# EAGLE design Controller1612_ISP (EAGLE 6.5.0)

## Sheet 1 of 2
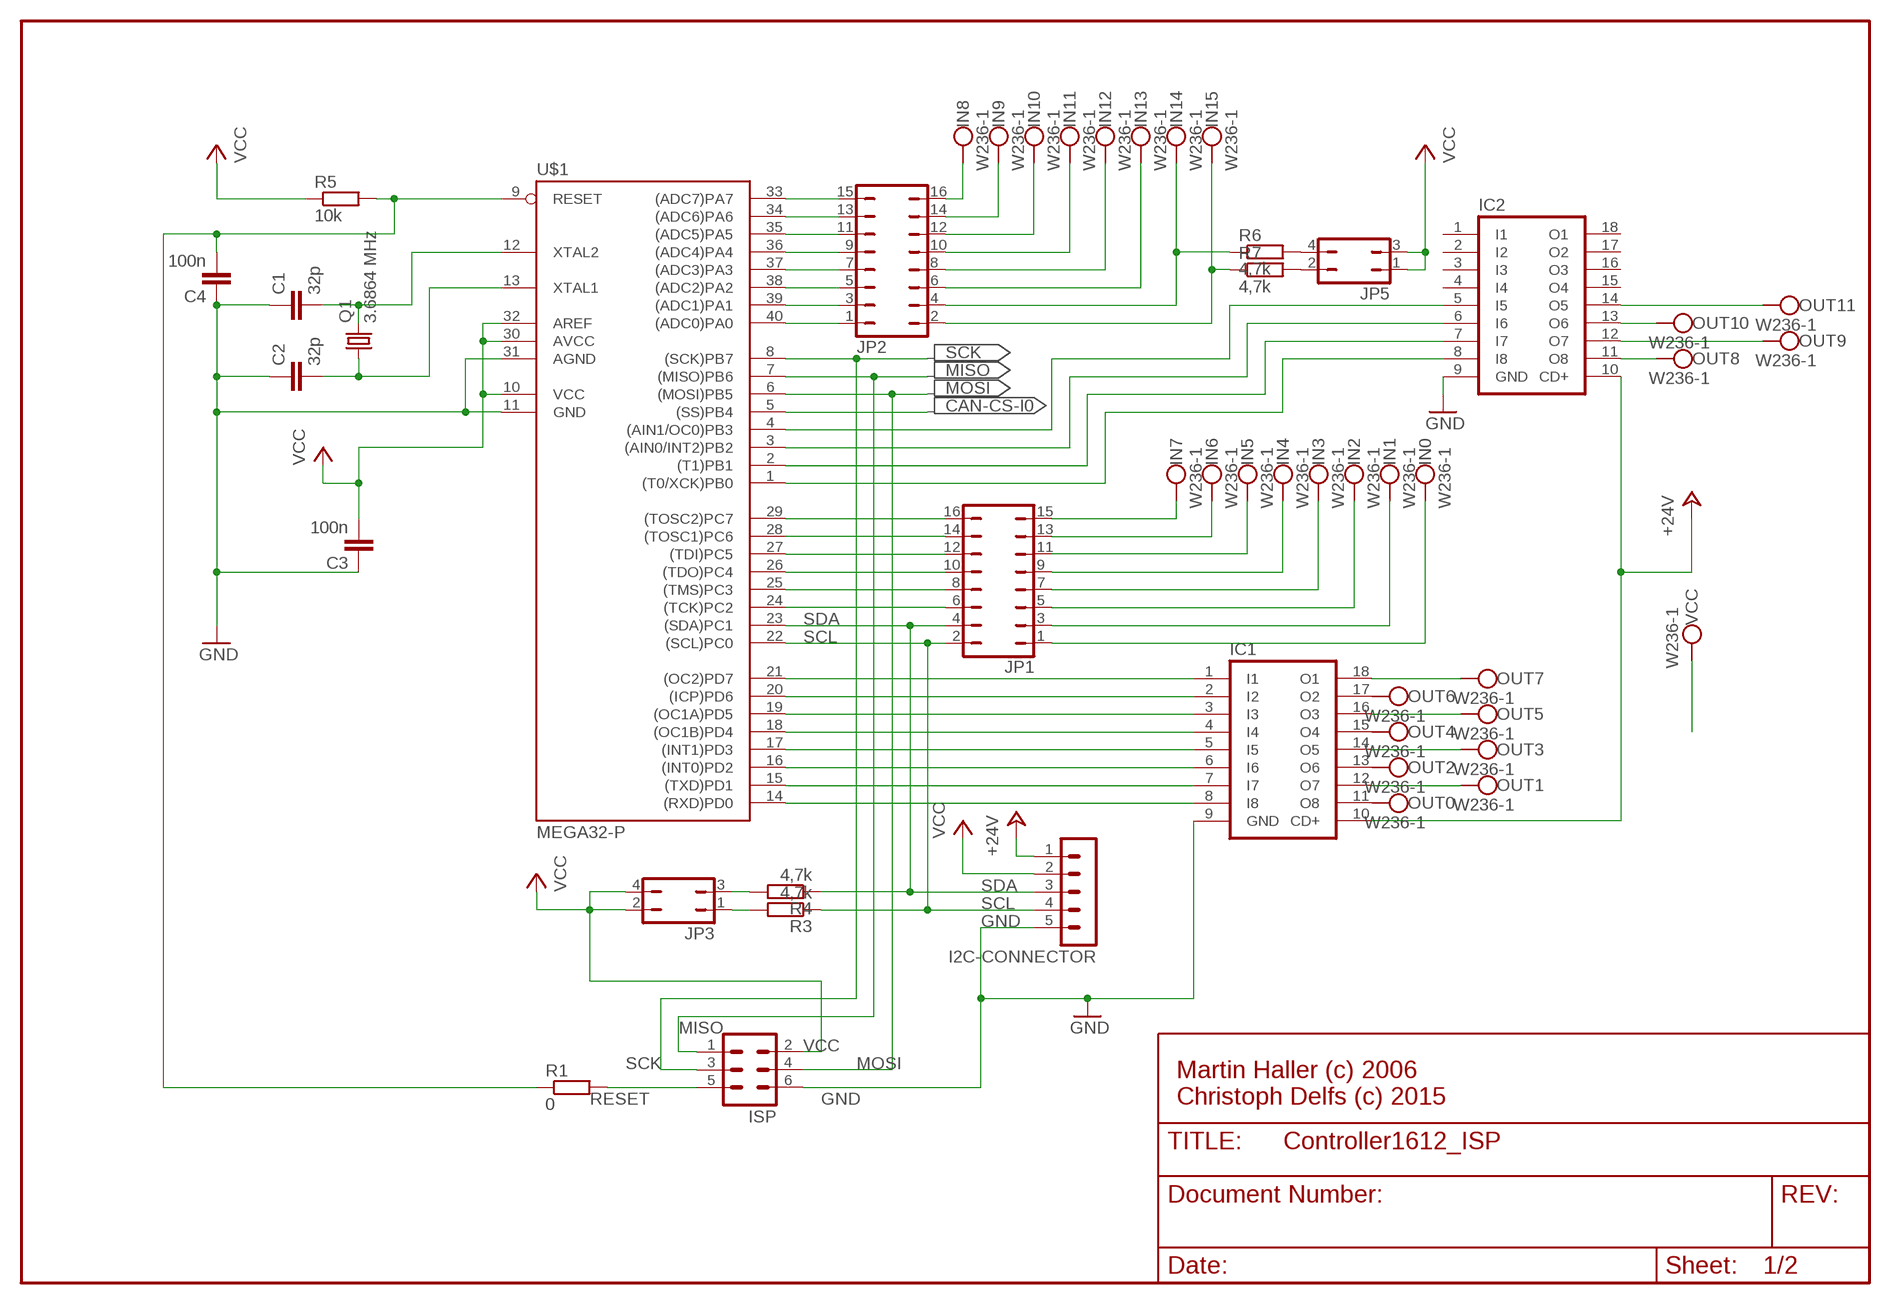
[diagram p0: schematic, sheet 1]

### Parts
C1  32p  C-EU025-024X044  [C025-024X044]
C2  32p  C-EU025-024X044  [C025-024X044]
C3  100n  C-EU050-025X075  [C050-025X075]
C4  100n  C-EU050-025X075  [C050-025X075]
I2C-CONNECTOR  MA05-1  [MA05-1]
IC1  ULN2803A  [DIL18]
IC2  ULN2803A  [DIL18]
IN0  W236-1  [W236-1]
IN1  W236-1  [W236-1]
IN2  W236-1  [W236-1]
IN3  W236-1  [W236-1]
IN4  W236-1  [W236-1]
IN5  W236-1  [W236-1]
IN6  W236-1  [W236-1]
IN7  W236-1  [W236-1]
IN8  W236-1  [W236-1]
IN9  W236-1  [W236-1]
IN10  W236-1  [W236-1]
IN11  W236-1  [W236-1]
IN12  W236-1  [W236-1]
IN13  W236-1  [W236-1]
IN14  W236-1  [W236-1]
IN15  W236-1  [W236-1]
ISP  ML6  [ML6]
JP1  JP8Q  [JP8Q]
JP2  JP8Q  [JP8Q]
JP3  JP2Q  [JP2Q]
JP5  JP2Q  [JP2Q]
OUT0  W236-1  [W236-1]
OUT1  W236-1  [W236-1]
OUT2  W236-1  [W236-1]
OUT3  W236-1  [W236-1]
OUT4  W236-1  [W236-1]
OUT5  W236-1  [W236-1]
OUT6  W236-1  [W236-1]
OUT7  W236-1  [W236-1]
OUT8  W236-1  [W236-1]
OUT9  W236-1  [W236-1]
OUT10  W236-1  [W236-1]
OUT11  W236-1  [W236-1]
Q1  3.6864 MHz  CRYTALHC49U70  [HC49U70]
R1  0  R-EU_0204/2V  [0204V]
R3  4,7k  R-EU_0204/7  [0204/7]
R4  4,7k  R-EU_0204/7  [0204/7]
R5  10k  R-EU_0207/12  [0207/12]
R6  4,7k  R-EU_0207/2V  [0207/2V]
R7  4,7k  R-EU_0207/2V  [0207/2V]
U$1  MEGA32-P  [DIL40]
VCC  W236-1  [W236-1]

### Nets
+24V: I2C-CONNECTOR.1 IC1.10(CD+) IC2.10(CD+) ; also sheet 2
CAN-CS-I0: U$1.5((SS)PB4) ; also sheet 2
GND: C1.1 C2.1 C3.1 C4.1 I2C-CONNECTOR.5 IC1.9(GND) IC2.9(GND) ISP.6 U$1.11(GND) U$1.31(AGND) ; also sheet 2
INPUT2: IN3.1(KL1) JP1.7
MISO: ISP.1 U$1.7((MISO)PB6) ; also sheet 2
MOSI: ISP.4 U$1.6((MOSI)PB5) ; also sheet 2
N$1: C1.2 Q1.2 U$1.12(XTAL2)
N$2: C2.2 Q1.1 U$1.13(XTAL1)
N$3: IN0.1(KL1) JP1.1
N$4: IN1.1(KL1) JP1.3
N$5: IN2.1(KL1) JP1.5
N$6: JP2.1 U$1.40((ADC0)PA0)
N$7: IN4.1(KL1) JP1.9
N$8: IN5.1(KL1) JP1.11
N$9: IN6.1(KL1) JP1.13
N$10: IN7.1(KL1) JP1.15
N$11: JP2.3 U$1.39((ADC1)PA1)
N$12: JP2.5 U$1.38((ADC2)PA2)
N$13: JP3.1 R3.2
N$14: JP2.7 U$1.37((ADC3)PA3)
N$15: JP2.9 U$1.36((ADC4)PA4)
N$16: JP2.11 U$1.35((ADC5)PA5)
N$17: JP2.13 U$1.34((ADC6)PA6)
N$18: IC1.1(I1) U$1.21((OC2)PD7)
N$19: IC1.2(I2) U$1.20((ICP)PD6)
N$20: IC1.3(I3) U$1.19((OC1A)PD5)
N$21: IC1.4(I4) U$1.18((OC1B)PD4)
N$22: IC1.5(I5) U$1.17((INT1)PD3)
N$23: IC1.6(I6) U$1.16((INT0)PD2)
N$24: IC1.7(I7) U$1.15((TXD)PD1)
N$25: IC1.8(I8) U$1.14((RXD)PD0)
N$26: IC1.11(O8) OUT0.1(KL1)
N$27: IC1.12(O7) OUT1.1(KL1)
N$28: IC1.13(O6) OUT2.1(KL1)
N$29: IC1.14(O5) OUT3.1(KL1)
N$30: IC1.15(O4) OUT4.1(KL1)
N$31: IC1.16(O3) OUT5.1(KL1)
N$32: IC1.17(O2) OUT6.1(KL1)
N$33: IC1.18(O1) OUT7.1(KL1)
N$34: IC2.8(I8) U$1.1((T0/XCK)PB0)
N$35: IC2.7(I7) U$1.2((T1)PB1)
N$36: IC2.6(I6) U$1.3((AIN0/INT2)PB2)
N$37: IC2.5(I5) U$1.4((AIN1/OC0)PB3)
N$38: IC2.11(O8) OUT8.1(KL1)
N$39: IC2.12(O7) OUT9.1(KL1)
N$40: IC2.13(O6) OUT10.1(KL1)
N$41: IC2.14(O5) OUT11.1(KL1)
N$42: JP2.15 U$1.33((ADC7)PA7)
N$52: IN8.1(KL1) JP2.16
N$53: IN9.1(KL1) JP2.14
N$54: IN10.1(KL1) JP2.12
N$55: IN11.1(KL1) JP2.10
N$56: IN12.1(KL1) JP2.8
N$57: IN13.1(KL1) JP2.6
N$58: IN14.1(KL1) JP2.4 R6.1
N$59: IN15.1(KL1) JP2.2 R7.1
N$60: JP3.3 R4.2
N$61: ISP.5 R1.2
N$62: JP1.6 U$1.24((TCK)PC2)
N$63: JP1.8 U$1.25((TMS)PC3)
N$64: JP1.10 U$1.26((TDO)PC4)
N$65: JP1.12 U$1.27((TDI)PC5)
N$66: JP1.14 U$1.28((TOSC1)PC6)
N$67: JP1.16 U$1.29((TOSC2)PC7)
N$68: JP5.4 R6.2
N$70: JP5.2 R7.2
RESET: C4.2 R1.1 R5.2 U$1.9(RESET)
SCK: ISP.3 U$1.8((SCK)PB7) ; also sheet 2
SCL: I2C-CONNECTOR.4 JP1.2 R3.1 U$1.22((SCL)PC0)
SDA: I2C-CONNECTOR.3 JP1.4 R4.1 U$1.23((SDA)PC1)
VCC: C3.2 I2C-CONNECTOR.2 ISP.2 JP3.2 JP3.4 JP5.1 JP5.3 R5.1 U$1.10(VCC) U$1.30(AVCC) U$1.32(AREF) VCC.1(KL1) ; also sheet 2
Unconnected: IC2.1(I1) IC2.2(I2) IC2.3(I3) IC2.4(I4) IC2.15(O4) IC2.16(O3) IC2.17(O2) IC2.18(O1) IN0.2(KL2) IN1.2(KL2) IN2.2(KL2) IN3.2(KL2) IN4.2(KL2) IN5.2(KL2) IN6.2(KL2) IN7.2(KL2) IN8.2(KL2) IN9.2(KL2) IN10.2(KL2) IN11.2(KL2) IN12.2(KL2) IN13.2(KL2) IN14.2(KL2) IN15.2(KL2) OUT0.2(KL2) OUT1.2(KL2) OUT2.2(KL2) OUT3.2(KL2) OUT4.2(KL2) OUT5.2(KL2) OUT6.2(KL2) OUT7.2(KL2) OUT8.2(KL2) OUT9.2(KL2) OUT10.2(KL2) OUT11.2(KL2) VCC.2(KL2)

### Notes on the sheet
- Martin Haller (c) 2006
  Christoph Delfs (c) 2015

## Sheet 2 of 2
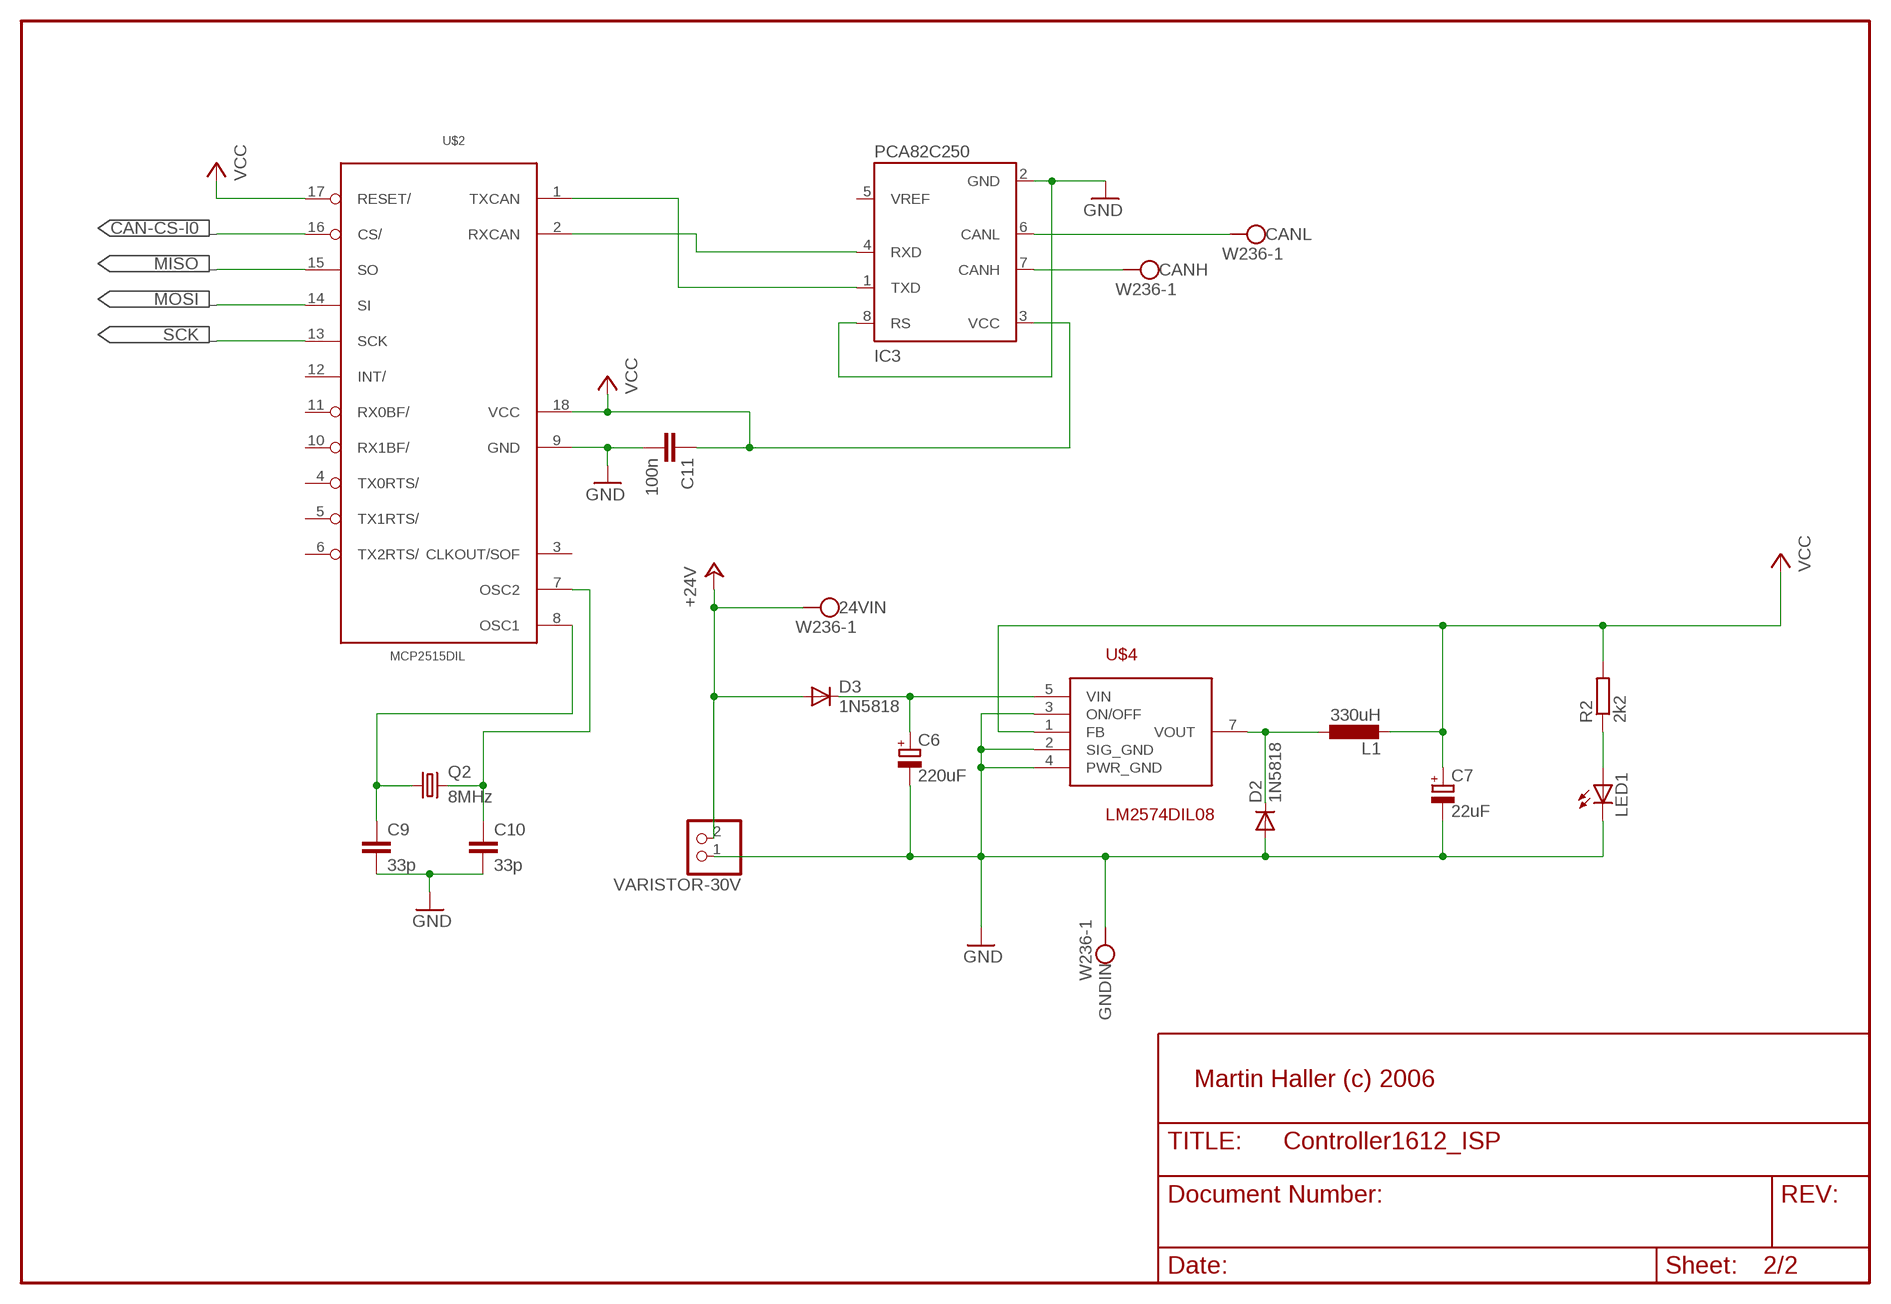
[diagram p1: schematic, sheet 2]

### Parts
24VIN  W236-1  [W236-1]
C6  220uF  CPOL-EUE22-10AXIAL  [E22-10]
C7  22uF  CPOL-EUE15-6AXIAL  [E15-6]
C9  33p  C-EU025-024X044  [C025-024X044]
C10  33p  C-EU025-024X044  [C025-024X044]
C11  100n  C-EU050-025X075  [C050-025X075]
CANH  W236-1  [W236-1]
CANL  W236-1  [W236-1]
D2  1N5818  1N4148  [DO35-10]
D3  1N5818  1N4148  [DO35-10]
GNDIN  W236-1  [W236-1]
IC3  PCA82C250  [DIL08]
L1  330uH  L-EU2200-12.7  [2200-12.7]
LED1  LED3MM  [LED3MM]
Q2  8MHz  CRYTALHC49U70  [HC49U70]
R2  2k2  R-EU_0207/2V  [0207/2V]
U$2  MCP2515DIL  [DIL18]
U$4  LM2574DIL08  [DIL08]
VARISTOR-30V  PINHD-1X2  [1X02]

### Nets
+24V: 24VIN.1(KL1) D3.A VARISTOR-30V.2 ; also sheet 1
CAN-CS-I0: U$2.16(CS/) ; also sheet 1
GND: C6.- C7.- C9.2 C10.2 C11.2 D2.A GNDIN.1(KL1) IC3.2(GND) IC3.8(RS) LED1.K(C) U$2.9(GND) U$4.2(SIG_GND) U$4.3(ON/OFF) U$4.4(PWR_GND) VARISTOR-30V.1 ; also sheet 1
MISO: U$2.15(SO) ; also sheet 1
MOSI: U$2.14(SI) ; also sheet 1
N$43: C6.+ D3.C U$4.5(VIN)
N$44: IC3.4(RXD) U$2.2(RXCAN)
N$45: IC3.1(TXD) U$2.1(TXCAN)
N$46: C9.1 Q2.1 U$2.8(OSC1)
N$47: C10.1 Q2.2 U$2.7(OSC2)
N$48: CANH.1(KL1) IC3.7(CANH)
N$49: CANL.1(KL1) IC3.6(CANL)
N$50: D2.C L1.1 U$4.7(VOUT)
N$51: LED1.A R2.1
SCK: U$2.13(SCK) ; also sheet 1
VCC: C7.+ C11.1 IC3.3(VCC) L1.2 R2.2 U$2.17(RESET/) U$2.18(VCC) U$4.1(FB) ; also sheet 1
Unconnected: 24VIN.2(KL2) CANH.2(KL2) CANL.2(KL2) GNDIN.2(KL2) IC3.5(VREF) U$2.3(CLKOUT/SOF) U$2.4(TX0RTS/) U$2.5(TX1RTS/) U$2.6(TX2RTS/) U$2.10(RX1BF/) U$2.11(RX0BF/) U$2.12(INT/)

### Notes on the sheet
- Martin Haller (c) 2006

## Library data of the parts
24VIN CANH CANL GNDIN IN0 IN1-IN15 OUT0 OUT1-OUT11 VCC = con-wago-508:W236-1: WAGO SREW CLAMP
C1-C4 C9-C11 = rcl:C-EU: CAPACITOR, European symbol
C6 C7 = rcl:CPOL-EU: POLARIZED CAPACITOR, European symbol
D2 D3 = diode:1N4148: DIODE
I2C-CONNECTOR = con-lstb:MA05-1: PIN HEADER
IC1 IC2 = uln-udn:ULN2803A: DRIVER ARRAY
IC3 = micro-philips:PCA82C250: CAN CONTROLLER INTERFACE
ISP = con-ml:ML6: HARTING; OC_FARNELL: unknown; OC_NEWARK: unknown
JP1 JP2 = jumper:JP8Q: JUMPER
JP3 JP5 = jumper:JP2Q: JUMPER
L1 = rcl:L-EU: INDUCTOR, European symbol
LED1 = led:LED: LED
Q1 Q2 = crystal:CRYTAL: CRYSTAL
R1 = resistor:R-EU_: RESISTOR, European symbol
R2-R7 = rcl:R-EU_: RESISTOR, European symbol
U$1 = avr:MEGA32-P: MICROCONTROLLER 32 Kbytes FLASH 2 Kbytes SRAM 1 Kbytes EEPROM USART 8-channel 10 bit ADC
U$2 = MCP2515_MT:MCP2515*: MCP2515 Standalone CAN-Controller by Microchip Eagle-Lib. by MartinThomas
U$4 = hausbus-bauteile:LM2574
VARISTOR-30V = pinhead:PINHD-1X2: PIN HEADER

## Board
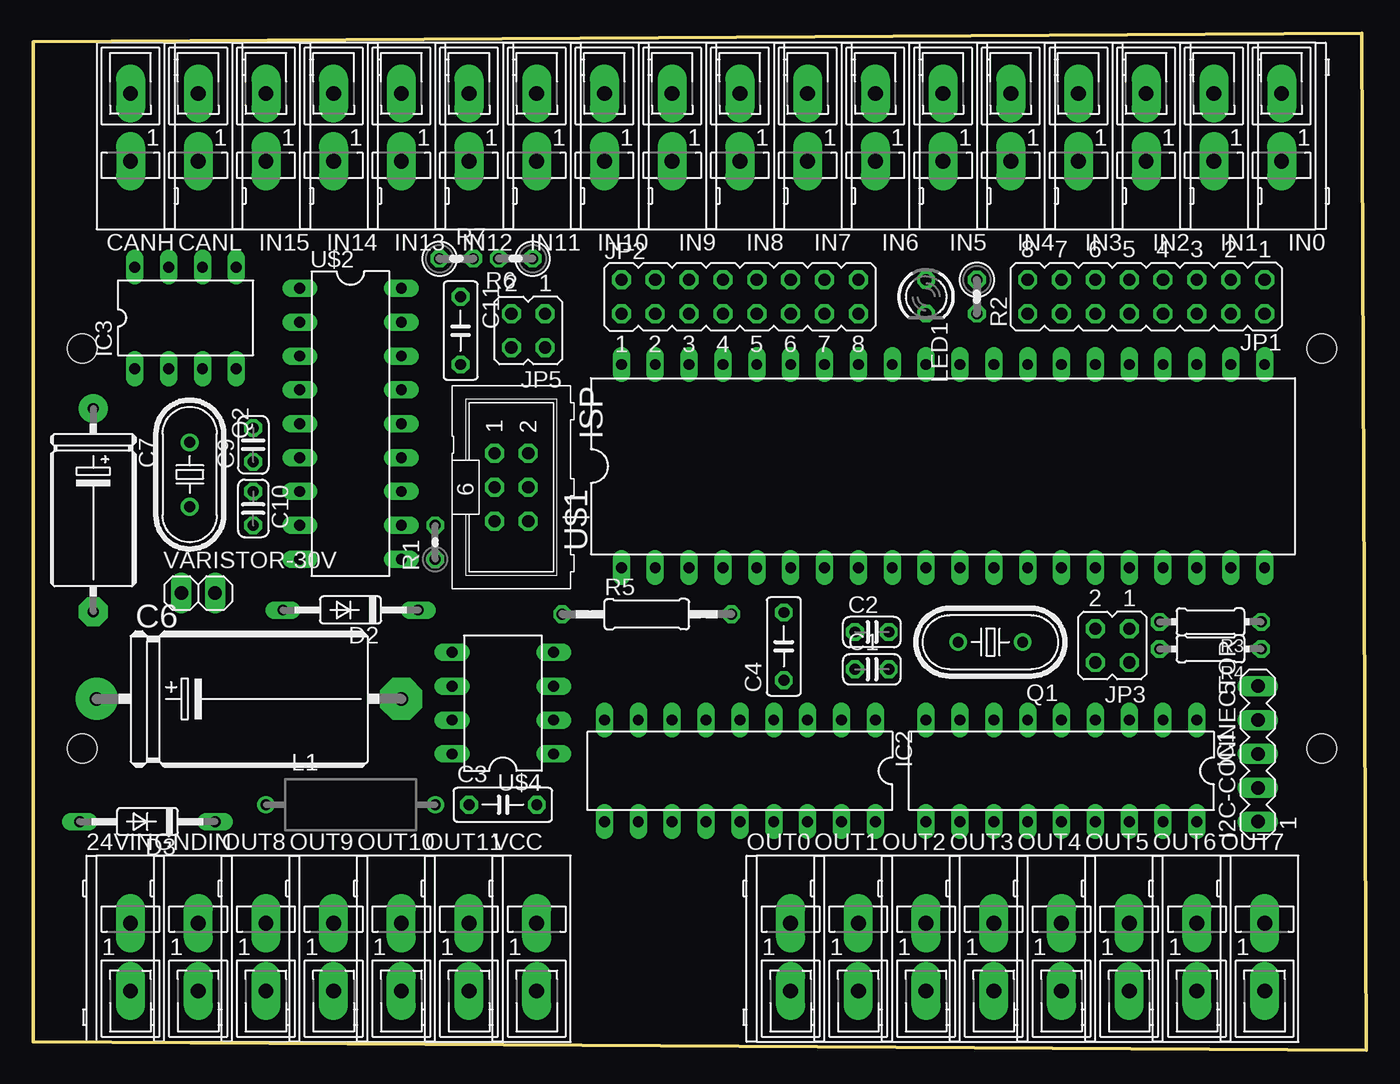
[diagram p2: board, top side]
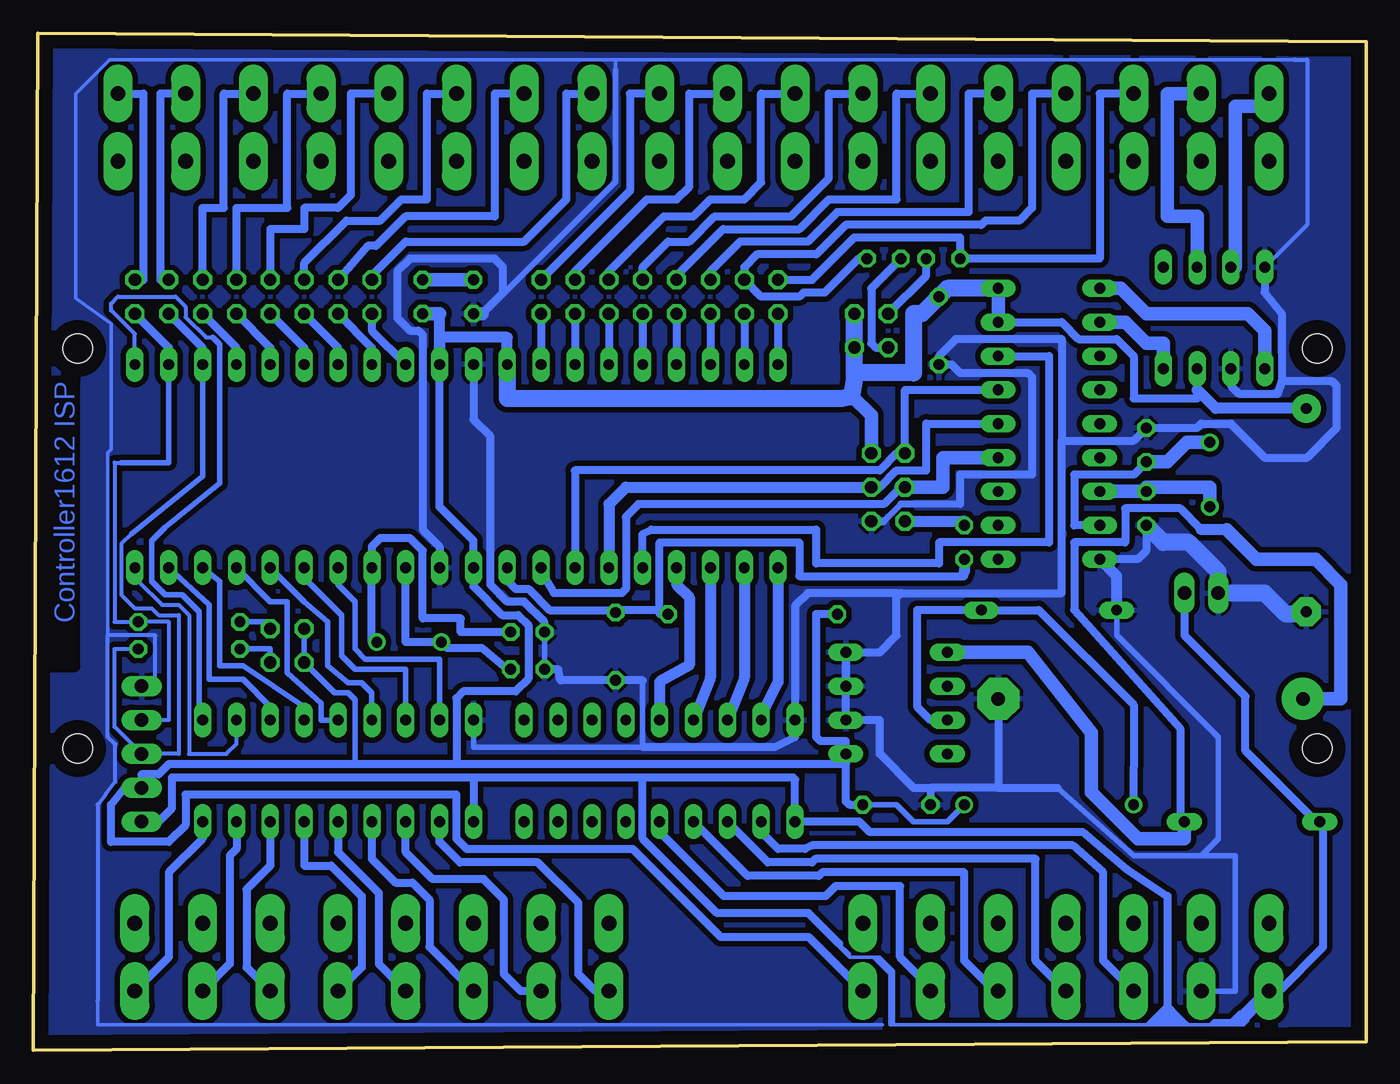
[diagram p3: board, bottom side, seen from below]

Size 100 x 76.27 mm. Coordinates in mm from the lower left corner, seen from the top.
Outline: 100,0 99.68,76.27 0,75.64 0,0.64 100,0
Copper layers (1*16): Top 0.035mm / dielectric 1.5mm / Bottom 0.035mm
Design rules "default": minimum track width 10mil, minimum drill 24mil, track to track 8mil, track to pad 8mil, pad to pad 8mil, via to via 8mil, smd to smd 8mil, copper to edge 40mil, drill to drill 8mil, minimum pad ring 10mil, minimum via ring 8mil, stop-mask expansion 4mil, vias tented up to drill 0mil, thermal gap 10mil
Holes 2.2 mm at 3.67,22.64 3.67,52.63 96.67,22.64 96.67,52.63

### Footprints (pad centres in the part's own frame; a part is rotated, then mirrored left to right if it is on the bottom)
W236-1 = drill 1.118 pad 2.184 long: 1 0,-2.54; 2 0,2.54
C025-024X044 = drill 0.813 octagon: 1 -1.27,0; 2 1.27,0
C050-025X075 = drill 0.813 octagon: 1 -2.54,0; 2 2.54,0
E22-10 = drill 1.016 pad 3.15: + -11.43,0 | drill 1.016 pad 3.15 octagon: - 11.43,0
E15-6 = drill 0.813 pad 2.159: + -7.62,0 | drill 0.813 pad 2.159 octagon: - 7.62,0
DO35-10 = drill 0.813 long: A 5.08,0; C -5.08,0
MA05-1 = drill 1.016 long: 1 -5.08,0; 2 -2.54,0; 3 0,0; 4 2.54,0; 5 5.08,0
DIL18 = drill 0.813 long: 1 -10.16,-3.81; 2 -7.62,-3.81; 3 -5.08,-3.81; 4 -2.54,-3.81; 5 0,-3.81; 6 2.54,-3.81; 7 5.08,-3.81; 8 7.62,-3.81; 9 10.16,-3.81; 10 10.16,3.81; 11 7.62,3.81; 12 5.08,3.81; 13 2.54,3.81; 14 0,3.81; 15 -2.54,3.81; 16 -5.08,3.81; 17 -7.62,3.81; 18 -10.16,3.81
DIL08 = drill 0.813 long: 1 -3.81,-3.81; 2 -1.27,-3.81; 3 1.27,-3.81; 4 3.81,-3.81; 5 3.81,3.81; 6 1.27,3.81; 7 -1.27,3.81; 8 -3.81,3.81
ML6 = drill 0.914 octagon: 1 -2.54,-1.27; 2 -2.54,1.27; 3 0,-1.27; 4 0,1.27; 5 2.54,-1.27; 6 2.54,1.27
JP8Q = drill 0.914 octagon: 1 -8.89,-1.27; 2 -8.89,1.27; 3 -6.35,-1.27; 4 -6.35,1.27; 5 -3.81,-1.27; 6 -3.81,1.27; 7 -1.27,-1.27; 8 -1.27,1.27; 9 1.27,-1.27; 10 1.27,1.27; 11 3.81,-1.27; 12 3.81,1.27; 13 6.35,-1.27; 14 6.35,1.27; 15 8.89,-1.27; 16 8.89,1.27
JP2Q = drill 0.914 octagon: 1 -1.27,-1.27; 2 1.27,-1.27; 3 -1.27,1.27; 4 1.27,1.27
2200-12.7 = drill 0.8 pad 1.27: 1 -6.35,0; 2 6.35,0
LED3MM = drill 0.813 octagon: A -1.27,0; K 1.27,0
HC49U70 = drill 0.813: 1 -2.413,0; 2 2.413,0
0204V = drill 0.813 octagon: 1 -1.27,0; 2 1.27,0
0207/2V = drill 0.813 octagon: 1 -1.27,0; 2 1.27,0
0204/7 = drill 0.813 octagon: 1 -3.81,0; 2 3.81,0
0207/12 = drill 0.813 octagon: 1 -6.35,0; 2 6.35,0
DIL40 = drill 0.813 long: 1 -24.13,-7.62; 2 -21.59,-7.62; 3 -19.05,-7.62; 4 -16.51,-7.62; 5 -13.97,-7.62; 6 -11.43,-7.62; 7 -8.89,-7.62; 8 -6.35,-7.62; 9 -3.81,-7.62; 10 -1.27,-7.62; 11 1.27,-7.62; 12 3.81,-7.62; 13 6.35,-7.62; 14 8.89,-7.62; 15 11.43,-7.62; 16 13.97,-7.62; 17 16.51,-7.62; 18 19.05,-7.62; 19 21.59,-7.62; 20 24.13,-7.62; 21 24.13,7.62; 22 21.59,7.62; 23 19.05,7.62; 24 16.51,7.62; 25 13.97,7.62; 26 11.43,7.62; 27 8.89,7.62; 28 6.35,7.62; 29 3.81,7.62; 30 1.27,7.62; 31 -1.27,7.62; 32 -3.81,7.62; 33 -6.35,7.62; 34 -8.89,7.62; 35 -11.43,7.62; 36 -13.97,7.62; 37 -16.51,7.62; 38 -19.05,7.62; 39 -21.59,7.62; 40 -24.13,7.62
1X02 = drill 1.016 long: 1 -1.27,0; 2 1.27,0

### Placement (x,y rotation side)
24VIN  7.29,6.98 0 top
C1  62.92,28.58 0 top
C2  62.92,31.37 0 top
C3  35.23,18.42 0 top
C4  56.31,30.29 90 top
C6  16.18,26.35 0 top
C7  4.5,40.51 270 top
C9  16.5,45.4 90 top
C10  16.5,40.64 270 top
C11  32.05,53.98 270 top
CANH  7.29,69.22 180 top
CANL  12.37,69.22 180 top
D2  23.8,33.02 180 top
D3  8.56,17.15 180 top
GNDIN  12.37,6.98 0 top
I2C-CONNECTOR  91.87,22.23 90 top
IC1  77.14,20.96 180 top
IC2  53.01,20.96 180 top
IC3  11.42,54.93 0 top
IN0  93.65,69.22 180 top
IN1  88.57,69.22 180 top
IN2  83.49,69.22 180 top
IN3  78.41,69.22 180 top
IN4  73.33,69.22 180 top
IN5  68.25,69.22 180 top
IN6  63.17,69.22 180 top
IN7  58.09,69.22 180 top
IN8  53.01,69.22 180 top
IN9  47.93,69.22 180 top
IN10  42.85,69.22 180 top
IN11  37.77,69.22 180 top
IN12  32.69,69.22 180 top
IN13  27.61,69.22 180 top
IN14  22.53,69.22 180 top
IN15  17.45,69.22 180 top
ISP  35.87,42.23 270 top
JP1  83.49,56.52 180 top
JP2  53.01,56.52 0 top
JP3  80.95,30.35 180 top
JP5  37.14,53.98 180 top
L1  23.8,18.42 0 top
LED1  66.98,56.52 270 top
OUT0  56.82,6.98 0 top
OUT1  61.9,6.98 0 top
OUT2  66.98,6.98 0 top
OUT3  72.06,6.98 0 top
OUT4  77.14,6.98 0 top
OUT5  82.22,6.98 0 top
OUT6  87.3,6.98 0 top
OUT7  92.38,6.98 0 top
OUT8  17.45,6.98 0 top
OUT9  22.53,6.98 0 top
OUT10  27.61,6.98 0 top
OUT11  32.69,6.98 0 top
Q1  71.81,30.61 180 top
Q2  11.73,43.18 270 top
R1  30.15,38.1 90 top
R2  70.79,56.52 270 top
R3  88.32,32.13 180 top
R4  88.32,30.1 180 top
R5  46.02,32.7 0 top
R6  36.18,59.37 180 top
R7  31.74,59.37 0 top
U$1  68.25,43.81 0 top
U$2  23.8,46.99 270 top
U$4  35.23,26.04 90 top
VARISTOR-30V  12.37,34.29 0 top
VCC  37.77,6.98 0 top

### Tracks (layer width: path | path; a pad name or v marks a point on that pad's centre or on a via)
+24V
  Bottom 0.254: 9.83,1.91 9.2,2.54 9.2,2.22 9.51,1.91 | 11.73,1.91 13.32,1.91 | 13.32,1.91 13.64,1.91 | 13.96,1.91 14.28,1.91 | 14.59,1.91 14.91,1.91 | 14.91,2.41 14.91,2.22 | 14.91,2.22 14.91,1.91 | 14.91,1.91 15.23,1.91 | 15.23,1.91 15.54,1.91 | 16.18,1.91 16.5,1.91 | 16.5,1.91 35.48,1.91 | 35.48,1.91 35.74,1.91 35.74,6.22 | 35.74,6.22 36.5,6.98 36.75,6.98 | 37.01,6.98 38.79,6.98 | 38.79,6.98 39.55,7.75 | 38.79,6.98 38.79,7.24 39.55,8 | 35.48,1.91 35.48,5.71 | 35.48,5.71 35.48,5.97 35.74,6.22 | 35.74,6.22 35.99,6.22 | 35.99,6.22 36.75,6.98 | 35.99,6.22 35.48,5.71 | 35.48,5.71 35.74,5.71 37.01,6.98 | 37.01,6.98 36.75,6.98 | 13.64,1.91 13.64,2.22 | 13.64,2.22 14.28,2.86 | 14.28,2.86 14.59,3.17 | 14.59,3.17 14.59,2.54 | 14.59,1.91 14.59,2.22 | 14.59,2.54 14.28,2.86 | 14.28,2.86 14.28,2.54 13.64,1.91 | 13.64,1.91 13.96,1.91 | 13.96,1.91 14.59,2.54 | 14.59,2.54 14.59,2.22 | 14.59,2.22 14.28,1.91 | 14.59,1.91 14.91,2.22 | 15.23,2.22 15.23,1.91 | 15.23,1.91 14.91,2.22 | 14.91,2.22 15.23,2.22 | 15.23,3.17 14.91,3.49 14.59,3.17 | 9.51,1.91 9.83,1.91 | 9.83,1.91 9.83,2.22 | 9.83,2.54 9.51,2.54 9.83,2.22 | 9.83,2.22 9.83,2.54 | 9.83,2.54 9.51,2.86 8.88,2.22 9.2,1.91 9.51,1.91 | 10.46,1.91 10.46,2.22 | 9.83,2.54 10.15,2.22 | 10.15,2.22 9.83,1.91 | 9.83,1.91 10.15,1.91 | 10.15,1.91 10.46,2.22 | 10.46,2.22 10.78,2.22 | 10.78,2.22 11.42,2.22 | 11.73,1.91 11.1,1.91 | 11.1,1.91 10.46,1.91 | 10.46,1.91 10.15,2.22 | 10.15,2.22 10.46,2.22 | 11.42,2.22 11.1,1.91 | 11.1,1.91 10.78,2.22 | 10.78,2.22 10.46,1.91 | 10.46,1.91 10.15,1.91 | 10.15,1.91 9.83,2.22 | 9.83,2.22 10.15,2.22 | 11.42,2.22 11.73,1.91 | 14.28,1.91 14.59,1.91 | 16.18,1.91 15.86,2.22 | 15.86,2.22 15.23,2.86 | 15.23,2.86 15.23,2.54 | 15.23,2.54 15.23,2.22
  Bottom 0.254: 15.23,2.22 15.54,1.91 | 15.54,1.91 15.86,2.22 | 15.86,2.22 15.54,2.22 15.23,2.54 | 15.23,2.86 15.23,3.17 | 15.23,3.17 16.5,1.91 | 16.18,1.91 15.54,1.91 | 14.91,2.22 14.59,2.54 | 13.64,2.22 13.32,1.91
  Bottom 0.61: 14.91,2.41 14.91,3.49 14.91,11.56 17.96,13.59 21.26,16.38 37.26,16.38 38.02,17.15 IC2.10 42.85,20.32 | 24VIN.1 6.53,4.45 3.23,7.75 3.23,16.89 D3.A 3.73,17.15 9.07,22.48 9.07,26.54 13.64,31.12 VARISTOR-30V.2 | 42.98,20.45 54.28,20.45 | 54.28,20.45 66.98,20.45 | 66.98,20.45 IC1.10 | 39.55,8 41.83,10.29 48.69,10.29 54.28,15.88 54.28,20.45 | 66.98,20.45 89.59,20.45 89.59,18.16 90.6,17.15 I2C-CONNECTOR.1
  Bottom 1.016: 24VIN.1 9.2,2.54
CAN-CS-I0
  Bottom 0.61: U$2.16 23.8,52.07 23.8,38.1 32.05,38.1 32.05,36.51 41.26,36.51 41.26,39.05 53.65,39.05 54.28,38.73 U$1.5
GND
  Bottom 0.254: 56.31,74.3 94.28,74.3 96.83,71.76 96.83,56.39 94.16,54.48 94.16,45.09 94.41,44.83 94.41,31.12 | 56.31,74.3 5.38,74.3 5.26,74.3 | 56.31,74.3 56.31,73.53 | 95.17,3.68 95.17,1.91 36.31,1.91
  Bottom 0.305: I2C-CONNECTOR.5 90.86,27.31 90.86,31.12 94.41,31.12 94.41,23.5 93.9,22.99 93.84,22.99 93.84,20.13 94.54,19.24 95.17,18.42 95.17,3.68 | 5.38,74.3 4.43,74.3 4.43,61.91 IC3.8
  Bottom 0.406: 23.17,19.69 17.45,14.61 12.37,14.61 | D2.A 18.72,31.12 11.1,23.5 11.1,15.88 12.37,14.61 | 12.37,14.61 9.83,14.61 9.83,4.45 GNDIN.1 | IC1.9 66.98,22.73 54.28,22.73 54.28,27.75 | C1.1 C2.1 | 56.31,73.53 56.31,65.15 66.22,55.24 LED1.K | 36.18,39.69 34.91,40.96
  Bottom 0.508: 30.47,40.96 34.91,40.96
  Bottom 0.61: U$4.2 36.5,24.77 36.5,22.23 33.96,19.69 32.69,19.69 | 54.28,22.73 44.37,22.73 42.85,23.5 IC2.9 42.85,33.34 41.9,34.29 35.23,34.29 35.23,33.97 | U$4.2 U$4.3 U$4.4 | 54.28,27.75 C4.1 60.44,27.75 60.63,28.58 C1.1 | 66.34,55.24 64.76,56.83 64.76,58.74 65.39,59.37 71.74,59.37 72.7,58.42 72.7,54.93 71.74,53.98 71.11,53.98 70.79,53.66 70.79,39.05 69.52,37.78 U$1.11 | 27.61,19.69 32.69,19.69 | 32.69,19.69 C3.1 | C6.- 27.61,19.69 | 27.61,19.69 23.17,19.69 | 6.34,50.16 2.53,50.16 2.21,49.85 2.21,46.67 4.43,44.45 7.61,44.45 10.15,46.99 12.37,46.99 12.69,46.67 C9.2 17.45,45.72 22.85,45.72 | 6.34,50.16 6.66,49.21 9.51,49.21 10.15,49.85 IC3.2 | IC3.8 7.61,56.83 6.34,55.24 6.34,50.16 | U$1.31 66.98,47.31 65.71,46.04 65.71,34.92 64.44,33.66 63.17,33.66 61.65,32.13 C2.1 | C10.2 16.5,37.46 17.13,36.83 U$2.9 | 22.85,45.72 22.85,53.34 30.79,53.34 32.05,52.07 C11.2 31.1,51.43 30.47,50.8 25.39,50.8 25.07,50.48 25.07,43.18 30.47,43.18 30.47,40.96 | 22.85,45.72 22.85,34.29 34.91,34.29 35.23,33.97 | 35.23,33.97 35.23,31.12 36.5,29.85 U$4.4 | U$4.2 U$4.4 | ISP.6 36.18,39.69
  Bottom 0.813: 19.04,36.83 U$2.9 18.72,35.56 D2.A
  Bottom 1.016: LED1.K 66.34,55.24
  Bottom 1.27: 4.31,32.7 6.02,32.7 7.61,34.29 VARISTOR-30V.1 11.1,35.88 13.32,38.1 15.23,38.1 C10.2
  pour Bottom (isolate 0.406): -0.33,75.57 99.68,76.2 100,0.64 -0.33,0.64
INPUT2
  Bottom 0.61: JP1.7 84.76,63.18 80.95,63.18 80.95,71.76 IN3.1
MISO
  Bottom 0.406: ISP.1 34.91,44.77
  Bottom 0.61: 34.91,44.77 35.23,44.77 36.5,43.5 59.36,43.5 U$1.7 | ISP.1 34.59,49.53 U$2.15
MOSI
  Bottom 0.61: ISP.4 36.5,42.23 35.23,43.5 33.01,43.5 33.01,46.99 U$2.14
  Bottom 0.813: U$1.6 56.82,40.96 55.55,42.23 ISP.4
N$1
  Bottom 0.61: U$1.12 72.06,30.61 Q1.2 68.95,30.16 66.34,30.16 64.44,28.58 C1.2
N$2
  Bottom 0.61: Q1.1 74.6,30.61 U$1.13 74.6,37.78 73.97,38.42 71.74,38.42 70.79,37.46 70.79,32.38 67.93,32.38 67.93,31.37 C2.2
N$3
  Bottom 0.61: IN0.1 91.75,71.76 91.75,57.78 JP1.1
N$4
  Bottom 0.61: IN1.1 90.48,71.76 90.48,57.78 JP1.3
N$5
  Bottom 0.61: JP1.5 87.3,63.18 85.71,63.18 85.71,71.76 IN2.1
N$6
  Bottom 0.61: JP2.1 U$1.40
N$7
  Bottom 0.61: IN4.1 76.19,71.76 76.19,64.14 77.14,63.18 79.68,63.18 79.68,61.59 82.22,61.59 JP1.9
N$8
  Bottom 0.61: JP1.11 79.68,59.05 76.5,62.23 73.97,62.23 72.38,63.82 70.47,63.82 70.47,71.76 IN5.1
N$9
  Bottom 0.61: IN6.1 65.39,71.76 65.39,62.55 72.06,62.55 74.28,60.32 74.92,60.32 JP1.13
N$10
  Bottom 0.61: JP1.15 74.6,58.1 72.06,60.64 63.17,60.64 60,63.82 60,71.76 IN7.1
N$11
  Bottom 0.61: JP2.3 U$1.39
N$12
  Bottom 0.61: JP2.5 U$1.38
N$13
  Bottom 0.406: R3.2 82.22,32.13 JP3.1
N$14
  Bottom 0.61: JP2.7 U$1.37
N$15
  Bottom 0.61: JP2.9 U$1.36
N$16
  Bottom 0.61: JP2.11 U$1.35
N$17
  Bottom 0.61: JP2.13 U$1.34
N$18
  Bottom 0.305: U$1.21 92.38,53.72 94.16,55.5 94.16,56.01 93.65,56.52 89.33,56.52 88.57,55.75 88.57,54.99 87.05,53.47 86.54,53.47
  Bottom 0.406: 86.54,53.47 86.03,52.96 86.03,42.54 90.09,39.24 91.11,38.23 91.11,35.18 90.09,34.16 88.82,34.16 87.55,32.89 87.55,25.02 IC1.1
N$19
  Bottom 0.305: 92.38,35.18 92.13,35.18 90.35,33.4 89.08,33.4 88.32,32.64 88.32,22.23 85.52,22.23 84.76,22.99 IC1.2
  Bottom 0.406: 92.38,35.18 U$1.20
N$20
  Bottom 0.406: IC1.3 82.22,25.78 84.25,27.81 86.79,27.81 86.79,33.4 U$1.19
N$21
  Bottom 0.406: IC1.4 79.68,25.78 84.25,28.83 86.03,28.83 86.03,35.18 U$1.18
N$22
  Bottom 0.406: IC1.5 78.41,24.77 78.41,26.04 80.95,28.32 80.95,33.66 82.22,33.66 U$1.17
N$23
  Bottom 0.406: IC1.6 74.6,26.8 75.36,27.56 76.38,27.56 77.9,28.83 77.9,32.13 79.68,33.66 U$1.16
N$24
  Bottom 0.406: U$1.15 79.68,35.43 76.89,32.64 76.89,29.59 75.87,28.58 72.06,28.58 IC1.7
N$25
  Bottom 0.406: IC1.8 69.52,29.34 75.11,29.34 75.87,30.1 75.87,33.66 77.14,34.92 U$1.14
N$26
  Bottom 0.61: OUT0.1 57.84,4.45 59.11,5.71 59.11,11.05 62.15,14.1 68,14.1 69.52,15.62 IC1.11
N$27
  Bottom 0.61: OUT1.1 63.42,4.45 64.69,5.71 64.69,11.3 66.22,12.83 70.03,12.83 72.06,14.86 IC1.12
N$28
  Bottom 0.61: IC1.13 74.6,14.35 72.82,12.57 71.55,12.57 70.28,11.3 70.28,7.75 OUT2.1
N$29
  Bottom 0.61: IC1.14 77.14,14.86 74.09,11.81 74.09,6.48 OUT3.1
N$30
  Bottom 0.61: IC1.15 79.68,13.84 77.65,13.84 75.36,11.56 75.36,6.22 OUT4.1
N$31
  Bottom 0.61: IC1.16 82.22,13.84 84,12.06 84,6.22 OUT5.1
N$32
  Bottom 0.61: IC1.17 84.76,15.11 85.27,14.61 85.27,6.48 OUT6.1
N$33
  Bottom 0.61: IC1.18 87.3,15.88 89.84,13.33 89.84,6.98 OUT7.1
N$34
  Bottom 0.813: U$1.1 44.12,27.62 45.39,25.08 IC2.8
N$35
  Bottom 0.813: U$1.2 46.66,27.94 IC2.7
N$36
  Bottom 0.813: U$1.3 49.2,27.94 IC2.6
N$37
  Bottom 0.813: U$1.4 51.74,34.92 50.79,33.97 50.79,28.89 53.01,27.62 IC2.5
N$38
  Bottom 0.61: IC2.11 45.39,16.38 44.12,15.11 42.09,15.11 41.58,15.37 22.02,15.37 19.74,13.33 19.74,6.73 OUT8.1
N$39
  Bottom 0.61: OUT9.1 24.82,6.73 24.82,14.35 41.33,14.35 41.58,14.1 44.88,14.1 IC2.12
N$40
  Bottom 0.61: OUT10.1 27.86,4.45 30.15,6.73 30.15,13.33 40.82,13.33 41.07,13.08 46.41,13.08 IC2.13
N$41
  Bottom 0.61: OUT11.1 32.69,4.7 34.98,6.98 34.98,12.32 39.8,12.32 40.56,11.56 48.18,11.56 53.01,16.38 IC2.14
N$42
  Bottom 0.61: JP2.15 U$1.33
N$43
  Bottom 0.61: 12.37,39.05 13.96,40.64 18.09,40.64 18.09,38.1 21.9,38.1 21.9,33.02 13.96,24.13 13.96,17.46 D3.C
  Bottom 0.813: 10.46,39.05 12.37,39.05
  Bottom 1.016: U$4.5 25.39,29.85 20.62,23.81 20.62,19.37 17.13,15.88 13.64,15.88 D3.C | C6.+ 1.89,26.35 1.89,34.92 3.8,36.83 8.24,36.83 10.46,39.05
N$44
  Bottom 1.016: U$2.2 18.09,54.61 16.5,53.02 15.23,53.02 IC3.4
N$45
  Bottom 1.016: U$2.1 18.4,57.15 16.5,55.24 8.88,55.24 7.61,53.98 IC3.1
N$46
  Bottom 0.61: C9.1 17.45,43.18 21.9,43.18 21.9,39.37 U$2.8
  Bottom 1.016: Q2.1 13.45,45.59 14.91,44.13 C9.1
N$47
  Bottom 1.016: U$2.7 C10.1 16.5,42.23 11.73,42.23 Q2.2
N$48
  Bottom 1.016: IC3.7 9.83,58.74 9.83,70.8 7.29,70.8 CANH.1
N$49
  Bottom 1.016: IC3.6 12.69,62.55 14.91,62.55 14.91,71.76 CANL.1
N$50
  Bottom 0.254: 17.45,20.96 17.45,21.21
  Bottom 0.61: L1.1 17.45,20.96 | 17.45,21.21 17.45,25.91 24.56,33.02 D2.C 33.71,33.02 33.71,25.78 32.69,24.77 U$4.7
N$51
  Bottom 1.016: LED1.A R2.1
N$52
  Bottom 0.61: IN8.1 55.23,71.76 55.23,64.45 JP2.16
N$53
  Bottom 0.61: JP2.14 59.36,58.42 53.96,63.82 51.74,63.82 50.79,64.77 50.79,71.76 IN9.1
N$54
  Bottom 0.61: JP2.12 56.82,58.42 52.69,62.55 50.47,62.55 49.2,63.82 46.66,63.82 45.39,65.09 45.39,71.76 IN10.1
N$55
  Bottom 0.61: JP2.10 54.28,58.74 52.38,60.64 50.79,60.64 48.88,62.55 43.17,62.55 40.31,65.41 40.31,71.76 IN11.1
N$56
  Bottom 0.61: JP2.8 51.74,58.1 48.25,61.59 42.53,61.59 40.31,63.82 35.23,63.82 35.23,71.76 IN12.1
N$57
  Bottom 0.61: IN13.1 29.83,71.76 29.83,62.86 39.68,62.86 41.9,60.64 46.98,60.64 49.2,58.42 JP2.6
N$58
  Bottom 0.61: IN14.1 25.07,71.76 25.07,63.18 26.02,62.23 28.56,62.23 28.88,61.91 39.04,61.91 41.26,59.69 45.71,59.69 46.66,58.74 JP2.4 45.39,56.52 42.53,56.52 42.22,56.83 40.63,56.83 38.09,59.37 R6.1
N$59
  Bottom 0.254: 30.15,59.69 R7.1
  Bottom 0.61: JP2.2 41.58,57.78 38.41,60.96 30.47,60.96 R7.1 19.99,59.37 19.99,71.76 IN15.1
N$60
  Bottom 0.406: R4.2 82.22,30.1 JP3.3
N$61
  Bottom 0.813: ISP.5 30.15,39.69 R1.2
N$62
  Bottom 0.61: U$1.24 84.76,52.7 JP1.6
N$63
  Bottom 0.61: U$1.25 82.22,52.7 JP1.8
N$64
  Bottom 0.61: U$1.26 79.68,52.7 JP1.10
N$65
  Bottom 0.61: U$1.27 77.14,52.7 JP1.12
N$66
  Bottom 0.61: U$1.28 74.6,52.7 JP1.14
N$67
  Bottom 0.61: JP1.16 74.6,53.98 U$1.29
N$68
  Bottom 0.61: R6.2 37.14,57.15 37.14,53.02 36.82,52.7 JP5.4
N$70
  Bottom 0.61: JP5.2 33.01,58.1 R7.2
RESET
  Bottom 0.61: 53.01,33.02 56.19,33.02 C4.2 56.44,33.02 61.27,33.02 62.85,34.61 63.81,34.61 64.44,35.24 U$1.9 | 53.01,33.02 R5.2 53.01,32.7 | 53.01,33.02 53.01,38.1 42.53,38.1 42.53,35.56 30.15,35.56 30.15,35.88
  Bottom 0.813: R1.1 30.15,35.88
SCK
  Bottom 0.61: U$1.8 61.9,35.88 60.95,34.29 55.87,34.29 55.55,34.61 55.55,40 54.6,40.96 36.18,40.96 34.91,42.23
  Bottom 1.016: U$2.13 31.74,44.45 31.74,42.23 ISP.3 34.91,42.23
SCL
  Bottom 0.305: 93.4,44.07 93.9,44.07 93.9,32.13 R3.1 89.84,32.13 89.84,24.77 I2C-CONNECTOR.4
  Bottom 0.406: 93.4,44.07 89.84,44.07 U$1.22
  Bottom 0.61: U$1.22 89.84,52.7 JP1.2
SDA
  Bottom 0.305: 92.63,38.73 93.4,37.97 93.4,34.16 92.38,33.15 91.11,33.15 90.6,32.64 89.08,32.64 89.08,22.23 I2C-CONNECTOR.3 93.9,24.26 93.9,30.1 R4.1
  Bottom 0.406: U$1.23 87.3,43.05 92.63,38.73
  Bottom 0.61: U$1.23 87.3,52.7 JP1.4
VCC
  Bottom 0.406: C3.2 35.23,18.42 33.96,17.15 31.42,17.15 L1.2 | 75.87,21.46 75.87,26.29 76.38,26.8 77.39,26.8 JP3.4 JP3.2
  Bottom 0.61: C3.2 38.79,18.42 39.04,18.67 39.04,21.46 | 39.04,21.46 U$4.1 39.04,23.18 40.95,23.18 41.26,23.5 41.26,32.7 R5.1 | 39.04,21.46 68.31,21.46 | 68.31,21.46 75.87,21.46 89.84,21.46 90.6,20.7 91.87,20.7 I2C-CONNECTOR.2 93.14,19.69 94.16,18.42 94.16,15.62 89.84,15.62 88.57,16.89 88.57,19.18 68.25,19.18 68.25,15.88 67.49,15.11 55.04,15.11 48.44,8.51 41.83,8.51 VCC.1 | U$1.30 69.52,40.77 66.98,38.23 U$1.10 66.98,34.8 64.82,32.64 63.61,32.64 62.85,31.88 62.85,27.88 63.81,26.92 67.74,26.92 68.25,26.42 68.25,21.53 68.31,21.46 | U$2.17 22.85,54.61 21.58,53.34 18.72,53.34 17.45,52.07 17.45,48.89 12.69,48.89 12.69,49.53 IC3.3
  Bottom 0.813: U$1.32 64.44,53.47 69.52,53.47 U$1.30 69.52,55.24 | C7.+ 11.29,48.13 12.69,49.53
  Bottom 1.016: 69.52,55.24 R2.2 | U$2.18 U$2.17 | ISP.2 37.14,47.62 38.56,49.05
  Bottom 1.27: U$2.18 31.42,57.15 C11.1 33.33,55.24 33.96,55.24 33.96,50.8 38.41,50.8 | 38.41,50.8 JP5.3 JP5.1 | U$1.32 64.44,48.89 39.36,48.89 38.56,49.05 38.41,50.16 38.41,50.8

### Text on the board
Bottom: Controller1612 ISP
